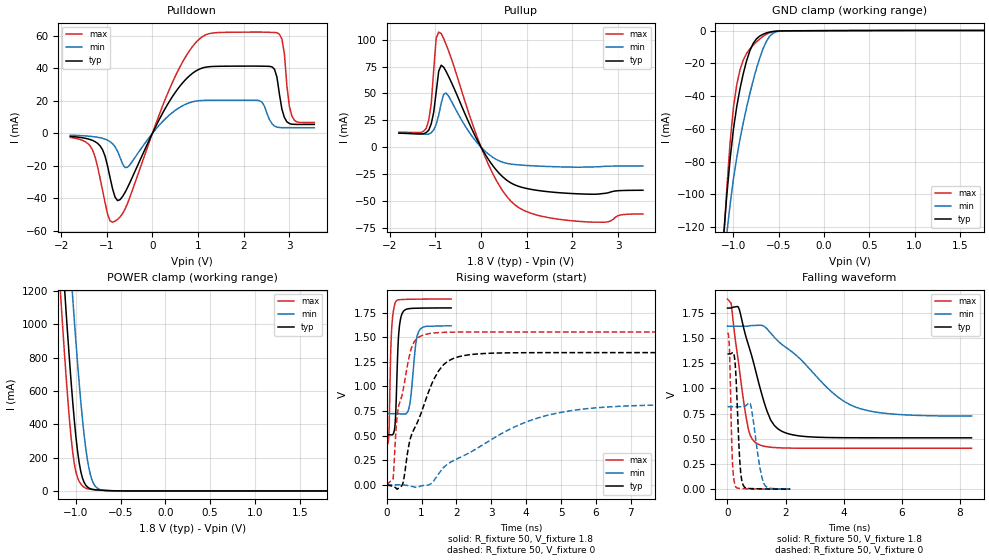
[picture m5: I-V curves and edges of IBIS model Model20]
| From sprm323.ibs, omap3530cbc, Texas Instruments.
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| Model based on original model for BQ0230CS_7LM
|   Sub model BQ0230CS_7LM_PD_ON_1P8
[model]   Model20
|[Input Load]   PD
|[Output Drive]
|Voltage   1.8V
|Mode   I/O
Model_type   I/O
Polarity   Non-Inverting
Enable   Active-Low
Vinl =  0.63
Vinh =  1.17
Cref =  15.0000pF
Rref =  100.0000M
Vref =  0V
Vmeas =  0.9
C_comp   0.6926437p   0.6051649p   0.8002447p
[Model Spec]
Vinl   0.63   0.567   0.6615
Vinh   1.17   1.053   1.2285
[Temperature Range]   25   125   -40
[Voltage Range]   1.8   1.62   1.89
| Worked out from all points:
|   slope of the pulldown table from 0 to 0.27 V, typ, clamps not added: 18.2 ohm
|   slope of the pullup table from 0 to 0.27 V, typ, clamps not added: 15.1 ohm
|   GND clamp passes 1 mA (typ) near -0.61 V on its own axis
|   POWER clamp passes 1 mA (typ) near -0.56 V on its own axis
|   rising waveform, R_fixture 50, V_fixture 1.8: 20-80 % time 82.8ps typ, 143ps min, 66.2ps max; typ from 0.51 V to 1.8 V
|   rising waveform, R_fixture 50, V_fixture 0: 20-80 % time 781ps typ, 2.51ns min, 384ps max; typ from 0 V to 1.34 V
|   falling waveform, R_fixture 50, V_fixture 1.8: 20-80 % time 760ps typ, 1.99ns min, 424ps max; typ from 1.8 V to 0.51 V
|   falling waveform, R_fixture 50, V_fixture 0: 20-80 % time 126ps typ, 249ps min, 80.4ps max; typ from 1.34 V to 0.001 V
[POWER_clamp]
-1.8V     7.03A      7.477A     6.772A
-1.182V   1.672A     2.34A      1.267A
-1.164V   1.518A     2.189A     1.114A
-1.127V   1.216A     1.889A     820.5mA
-1.073V   791.2mA    1.448A     431.2mA
-1.036V   538.2mA    1.164A     234.6mA
-963.6mV  169mA      647.7mA    57.37mA
-909.1mV  52.03mA    338.6mA    22.22mA
-872.7mV  24.23mA    189.8mA    13.46mA
-818.2mV  9.921mA    62.61mA    8.619mA
-709.1mV  3.907mA    5.01mA     3.883mA
1.8V      125.3uA    51.98uA    219uA
[Pulldown]
-1.8V     -1.896mA   -1.14mA    -2.549mA
-1.364V   -3.858mA   -1.868mA   -7.811mA
-1.145V   -7.758mA   -2.749mA   -27.9mA
-818.2mV  -39.37mA   -8.281mA   -54.21mA
-545.5mV  -33.49mA   -20.95mA   -43.25mA
654.5mV   30.89mA    16.9mA     43.68mA
1.418V    41.32mA    20.41mA    62.11mA
2.345V    41.43mA    20.12mA    62.44mA
2.618V    40.99mA    5.968mA    62.24mA
2.782V    24.07mA    3.525mA    61.09mA
3.055V    5.586mA    3.449mA    10.68mA
3.545V    5.467mA    3.446mA    6.63mA
[Pullup]
-1.8V     13mA       13.47mA    13.94mA
-1.2V     13.58mA    11.97mA    17.52mA
-1.091V   21.69mA    13.4mA     40.45mA
-1.036V   32.56mA    16.02mA    72.07mA
-981.8mV  51.55mA    21.35mA    101.5mA
-927.3mV  70.65mA    29.73mA    107.1mA
-818.2mV  74.4mA     49.19mA    101mA
-763.6mV  70.3mA     50.34mA    95.36mA
54.55mV   -4.057mA   -2.362mA   -5.698mA
709.1mV   -34.52mA   -16.04mA   -52.48mA
2.127V    -43.43mA   -18.65mA   -69mA
3.545V    -40.12mA   -17.52mA   -62.13mA
[GND_clamp]
-1.8V     -750.7mA   -623.3mA   -941.3mA
-1.109V   -125.7mA   -143.5mA   -129.9mA
-1.073V   -100.4mA   -123.9mA   -96.51mA
-1.036V   -78.32mA   -106.2mA   -68.27mA
-1V       -60.38mA   -90.77mA   -47.15mA
-963.6mV  -46.54mA   -77.63mA   -33.2mA
-890.9mV  -26.21mA   -56.2mA    -17.88mA
-818.2mV  -12.24mA   -38.36mA   -11.11mA
-709.1mV  -3.293mA   -16.65mA   -5.049mA
-600mV    -851.2uA   -3.412mA   -1.264mA
-490.9mV  -193.3uA   -326.3uA   -232.3uA
1.764V    125uA      52.52uA    217.2uA
[Ramp]
dV/dt_f   0.782654/0.7672619n  0.5430258/2.01801n   0.9032563/0.4288973n
dV/dt_r  0.8333443/0.7823102n  0.5074551/2.536065n   0.9659701/0.3847111n
R_load = 50
[Rising Waveform]
R_fixture = 50
V_fixture = 1.8
V_fixture_min = 1.62
V_fixture_max = 1.89
0s        510.1mV    723.2mV    406.6mV
66ps      510mV      723.2mV    529.1mV
114ps     508.6mV    723.4mV    1.317V
142ps     507.3mV    723.4mV    1.573V
254ps     681.2mV    723.4mV    1.859V
344ps     1.528V     722.5mV    1.881V
442ps     1.74V      719.9mV    1.883V
664ps     1.792V     821mV      1.886V
920ps     1.796V     1.561V     1.888V
1.848ns   1.798V     1.616V     1.888V
[Rising Waveform]
R_fixture = 50
V_fixture = 0
V_fixture_min = 0
V_fixture_max = 0
0s        195.2nV    87.26nV    423.3nV
186ps     -15.38mV   13.61uV    61.22mV
308ps     -44.01mV   178.9uV    718.2mV
468ps     19.72mV    -321.8uV   955.7mV
646ps     421.5mV    -10.82mV   1.304V
1.018ns   760.1mV    -8.534mV   1.518V
1.49ns    1.159V     112.4mV    1.547V
2.18ns    1.312V     291.2mV    1.553V
5.066ns   1.344V     741mV      1.553V
9.836ns   1.344V     816.1mV    1.553V
[Falling Waveform]
R_fixture = 50
V_fixture = 1.8
V_fixture_min = 1.62
V_fixture_max = 1.89
0s        1.799V     1.619V     1.888V
126ps     1.799V     1.619V     1.847V
364ps     1.811V     1.619V     1.29V
682ps     1.469V     1.619V     649.3mV
1.004ns   1.135V     1.627V     455.3mV
1.488ns   686mV      1.55V      416.6mV
2.108ns   549.1mV    1.388V     408.3mV
3.598ns   512.4mV    962.8mV    406.6mV
4.414ns   510.6mV    814.4mV    406.6mV
8.396ns   510.1mV    726.5mV    406.6mV
[Falling Waveform]
R_fixture = 50
V_fixture = 0
V_fixture_min = 0
V_fixture_max = 0
0s        1.344V     819.4mV    1.553V
66ps      1.344V     819.5mV    1.401V
144ps     1.35V      819.1mV    481.2mV
174ps     1.356V     818.9mV    249.2mV
266ps     1.238V     818.5mV    32.93mV
422ps     283.5mV    818.1mV    7.943mV
530ps     47.02mV    819.7mV    5.925mV
784ps     6.197mV    850mV      2.125mV
1.272ns   2.148mV    45.34mV    814uV
2.158ns   853.6uV    3.245mV    124.7uV
